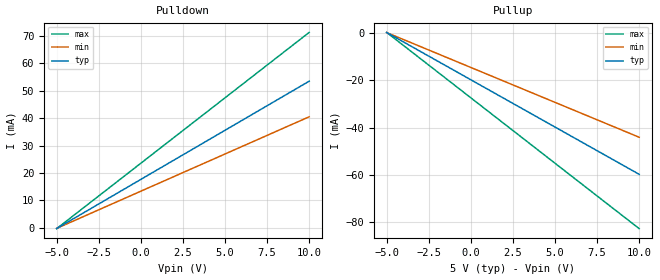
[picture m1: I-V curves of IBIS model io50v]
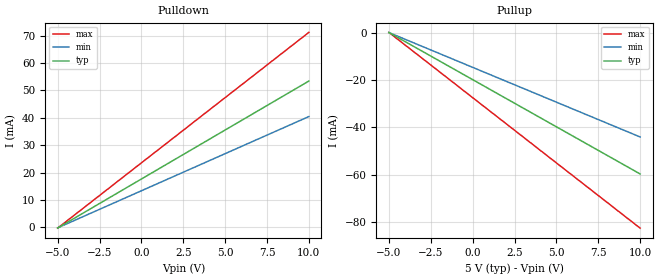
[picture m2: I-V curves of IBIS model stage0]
|********************* IBIS GOLDEN PARSER BUG REPORT FORM *********************
|INSTRUCTIONS
|To report a bug in the IBIS golden parser.  Please fill out the top part
|of the following form and send the complete form to ibischk-bug@vhdl.org.
|A list of reported bugs will be maintained on vhdl.org.
|PARSER VERSION NUMBER: 3.2.8
|PLATFORM (SPARC, HP700, PC, etc.): PC
|OS AND VERSION: Windows2000
|REPORTED BY: Arpad Muranyi
|DATE: 12/04/2001
|DESCRIPTION OF BUG:
|If all four delay numbers under the [Driver Schedule] keyword exist on
|one line, the parser issues an error.  This is in direct conflict with
|the IBIS specification, which says:
||   There are only five valid combinations in
||   which these delay values can be defined:
||   1)  Rise_on_dly   with   Fall_on_dly
||   2)  Rise_off_dly   with   Fall_off_dly
||   3)  Rise_on_dly   with   Rise_off_dly
||   4)  Fall_on_dly   with   Fall_off_dly
||   5)  All four delays defined
|IBISCHK3 V3.2.8
|Checking lab1sch.ibs for IBIS 3.2 Compatibility...
|ERROR (line   50) - Rise_on_dly and Fall_off_delay cannot be specified together
|ERROR (line   50) - Rise_off_dly and Fall_on_delay cannot be specified together
|WARNING - Model 'io50v': The [Driver_Schedule] has only one model defined
|Errors  : 2
|Warnings: 1
|File Failed
|INSERT IBIS FILE DEMONSTRATING THE BUG:
[IBIS Ver]   3.2
[File name]   bug64.ibs
[File rev]   0.00
[Date]   12/04/2001
[Source]   From silicon level SPICE model at Intel Corporation.
[Notes]   The following information corresponds to no chip.
[Disclaimer]   This information is for teaching purposes only.
[Component]   LAB_1
[Manufacturer]  Intel Corporation
[Package]
|   typ   min   max
R_pkg   50.000mOhm   40.000mOhm   60.000mOhm
L_pkg   5.00nH   4.00nH   6.00nH
C_pkg   2.00pF   1.00pF   3.00pF
[PIN]   signal_name   model_name   R_pin   L_pin   C_pin
1   Vcc   Power
2   GND   GND
7   Data_IO5_0   io50v
| Models and submodels in the file (2): io50v (I/O), stage0 (I/O)
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[Model]   io50v
Model_type   I/O
Vinl = 800.000mV
Vinh = 2.000V
Vmeas = 1.500V
Cref = 0.000F
|   typ   min   max
C_comp   4.550pF   2.600pF   6.500pF
[Voltage Range]   5.000V   4.750V   5.250V
[Temperature Range]   50.0   100.0   0.0
| Typical
[Driver Schedule]
| Model_Name   Rise_on_dly   Rise_off_dly   Fall_on_dly   Fall_off_dly
  stage0   0.000ns   10.000ns   0.000ns   10.000ns
  stage0   0.000ns   10.000ns   0.000ns   NA
  stage0   0.000ns   10.000ns   NA   10.000ns
  stage0   0.000ns   10.000ns   NA   NA
  stage0   0.000ns   NA   0.000ns   10.000ns
  stage0   0.000ns   NA   0.000ns   NA
  stage0   0.000ns   NA   NA   10.000ns
  stage0   0.000ns   NA   NA   NA
  stage0   NA   10.000ns   0.000ns   10.000ns
  stage0   NA   10.000ns   0.000ns   NA
  stage0   NA   10.000ns   NA   10.000ns
  stage0   NA   10.000ns   NA   NA
  stage0   NA   NA   0.000ns   10.000ns
  stage0   NA   NA   0.000ns   NA
  stage0   NA   NA   NA   10.000ns
  stage0   NA   NA   NA   NA
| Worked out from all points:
|   slope of the pulldown table from 0 to 0.75 V, typ, clamps not added: 280 ohm
|   slope of the pullup table from 0 to 0.75 V, typ, clamps not added: 251 ohm
[Pulldown]
|   Voltage   I(typ)   I(min)   I(max)
-5V       -207uA     -165.8uA   -256uA
10V       53.44mA    40.48mA    71.2mA
[Pullup]
|   Voltage   I(typ)   I(min)   I(max)
-5V       149.7uA    118uA      189.4uA
10V       -59.71mA   -44.06mA   -82.63mA
[Ramp]
R_load = 50.00Ohm
|   typ   min   max
dV/dt_r   1.403V/1.244ns   1.073V/1.741ns   1.793V/841.745ps
dV/dt_f   1.513V/1.302ns   1.150V/1.781ns   1.923V/870.817ps
[Model]   stage0
Model_type   I/O
Vinl = 800.000mV
Vinh = 2.000V
Vmeas = 1.500V
Cref = 0.000F
|   typ   min   max
C_comp   4.550pF   2.600pF   6.500pF
[Voltage Range]   5.000V   4.750V   5.250V
[Temperature Range]   50.0   100.0   0.0
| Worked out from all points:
|   slope of the pulldown table from 0 to 0.75 V, typ, clamps not added: 280 ohm
|   slope of the pullup table from 0 to 0.75 V, typ, clamps not added: 251 ohm
[Pulldown]
|   Voltage   I(typ)   I(min)   I(max)
-5V       -207uA     -165.8uA   -256uA
10V       53.44mA    40.48mA    71.2mA
[Pullup]
|   Voltage   I(typ)   I(min)   I(max)
-5V       149.7uA    118uA      189.4uA
10V       -59.71mA   -44.06mA   -82.63mA
[Ramp]
R_load = 50.00Ohm
|   typ   min   max
dV/dt_r   1.403V/1.244ns   1.073V/1.741ns   1.793V/841.745ps
dV/dt_f   1.513V/1.302ns   1.150V/1.781ns   1.923V/870.817ps
